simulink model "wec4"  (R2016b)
settings: Solver=ode4  StartTime=0  StopTime=1000  FixedStep=0.005  MaxStep=0.005  RelTol=1e-3  EnableMultiTasking=on
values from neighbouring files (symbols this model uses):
  arAdaptiveLawData = 1/2*zModelSimple.zModelPto.arFreq.*     zModelSimple.zModelPto.arMagnitude./     cos(zModelSimple.zModelPto.arPhase*pi/180+pi/2)    [IMPACT_Control.m]
  arAdaptiveLawDataX = 1/2*zModelSimpleX.zModelPto.arFreq.*         zModelSimpleX.zModelPto.arMagnitude./         cos(zModelSimpleX.zModelPto.arPhase*pi/180+pi/2)    [IMPACT_Control.m]
  arControllerRampGain = [0,0,1,1]    [IMPACT_Control.m]
  arControllerRampTime = [0 rStartRampTime rStartRampTime+rRampTimeLength 8000]    [IMPACT_Control.m]
  arEkfInitialisation = zeros(1,11)    [IMPACT_Control.m]
  arEkfInitialisationX = zeros(1,11)    [IMPACT_Control.m]
  arFrequency = zModelSimple.zModelPto.arFreq    [IMPACT_Control.m]
  arFrequencyRange = zModelSimple.zModelPto.arFreq    [IMPACT_Control.m]
  arFrequencyX = zModelSimpleX.zModelPto.arFreq    [IMPACT_Control.m]
  arImpedance = 1./zModelSimple.zModelPto.arMagnitude./zModelSimple.zModelPto.arFreq    [IMPACT_Control.m]
  arImpedanceX = 1./zModelSimpleX.zModelPto.arMagnitude./zModelSimpleX.zModelPto.arFreq    [IMPACT_Control.m]
  CentralPTOPreload = -1.6113e+07    (= -16113000)    [wecSimInputFile.m]
  F1 = [4.243 2.375 -12.243]    [wecSimInputFile.m]
  F2 = [4.243 -2.375 -12.243]    [wecSimInputFile.m]
  F3 = [-4.243 -2.375 -12.243]    [wecSimInputFile.m]
  F4 = [-4.243 2.375 -12.243]    [wecSimInputFile.m]
  FC = [0 0 -14]    [wecSimInputFile.m]
  iAdaptiveDamping = 0    [wec4IMPACT_Project.m]    (also in IMPACT_Control.m = handles.iAdaptiveDamping; wec1_IMPACT_Project.m; wec2_IMPACT_Project.m; wec3_IMPACT_Project.m)
  iControlType = 2    [wec4IMPACT_Project.m]    (also in IMPACT_Control.m = handles.iControlType; wec1_IMPACT_Project.m = 1; wec2_IMPACT_Project.m = 1; wec3_IMPACT_Project.m = 1)
  iPtoPositionConstraint = 1    [wec4IMPACT_Project.m]    (also in IMPACT_Control.m = handles.iPtoPositionConstraint; wec1_IMPACT_Project.m = 0; wec2_IMPACT_Project.m; wec3_IMPACT_Project.m)
  iSensorNoise = 0    [IMPACT_Control.m]
  m = m+1    (= 2)    [checkParamFile.m]
  PTOrotation = atan((T1(2)-F1(2))/(T1(1)-F1(1)))    [wecSimInputFile.m]
  rCogFloater = -8    [wec4_IMPACT_Model.m]    (also in paramInitial.m = get( handles.edit_rCogFloater, 'String' ); wec1_IMPACT_Model.m = -18; wec2_IMPACT_Model.m = -8.5; wec3_IMPACT_Model.m = -0.7)
  rCogSpar = -36.6    [wec4_IMPACT_Model.m]    (also in paramInitial.m = get( handles.edit_rCogSpar, 'String' ); wec3_IMPACT_Model.m = -21.3; wec3_IMPACT_Model2.m = -21.3)
  rDisplacementLimit = 10.000000    (= 10)    [wec4IMPACT_Project.m]    (also in IMPACT_Control.m = getValue(handles.edit_displacementLimit); wec1_IMPACT_Project.m; wec2_IMPACT_Project.m; wec3_IMPACT_Project.m = 3)
  rDisplacementLimitX = 10.000000    (= 10)    [wec4IMPACT_Project.m]    (also in IMPACT_Control.m = getValue(handles.edit_displacementLimitX); wec1_IMPACT_Project.m = 0; wec2_IMPACT_Project.m; wec3_IMPACT_Project.m = 0)
  rGainForAntiWIndUp = tfControllerDiscrete.rGain    [IMPACT_Control.m]
  rGainForAntiWIndUpX = tfControllerXDiscrete.rGain    [IMPACT_Control.m]
  rMaxForcePto = 300000000.000000    (= 300000000)    [wec4IMPACT_Project.m]    (also in IMPACT_Control.m = getValue(handles.edit_maxForcePto); wec1_IMPACT_Project.m = 1e+15; wec2_IMPACT_Project.m = 1e+15; wec3_IMPACT_Project.m = 1000000000)
  rMinForcePto = -300000000.000000    (= -300000000)    [wec4IMPACT_Project.m]    (also in IMPACT_Control.m = getValue(handles.edit_minForcePto); wec1_IMPACT_Project.m = -1e+15; wec2_IMPACT_Project.m = -1e+15; wec3_IMPACT_Project.m = -1000000000)
  rMooringX = 20000    [wec4_IMPACT_Model.m]    (also in paramInitial.m = get( handles.edit_rMooringX, 'String' ); wec3_IMPACT_Model.m = 10000; wec3_IMPACT_Model2.m = 10000)
  rMooringZ = 10000    [wec4_IMPACT_Model.m]    (also in paramInitial.m = get( handles.edit_rMooringZ, 'String' ); wec3_IMPACT_Model.m = 0; wec3_IMPACT_Model2.m = 0)
  rOutputSampleTime = 0.010000    (= 0.01)    [wec4IMPACT_Project.m]    (also in IMPACT_Control.m = getValue(handles.edit_outputSampleTime); wec1_IMPACT_Project.m; wec2_IMPACT_Project.m; wec3_IMPACT_Project.m)
  rPassiveDampingGain = -604830.000000    (= -604830)    [wec4IMPACT_Project.m]    (also in IMPACT_Control.m = getValue(handles.edit_gainPLD); wec1_IMPACT_Project.m = -214018.1537; wec2_IMPACT_Project.m = -1948070; wec3_IMPACT_Project.m = -519390)
  rPassiveDampingGainX = -278660.000000    (= -278660)    [wec4IMPACT_Project.m]    (also in IMPACT_Control.m = getValue(handles.edit_gainPLDX); wec1_IMPACT_Project.m = 0; wec2_IMPACT_Project.m = 0; wec3_IMPACT_Project.m = 0)
  rTetherPretension = 1.6113e+07    (= 16113000)    [wec4_IMPACT_Model.m]    (also in paramInitial.m = get( handles.edit_rTetherPretension, 'String' ); wec3_IMPACT_Model.m = 0; wec3_IMPACT_Model2.m = 0)
  rTetherSpring = 500000    [wec4_IMPACT_Model.m]    (also in paramInitial.m = get( handles.edit_rTetherSpring, 'String' ); wec3_IMPACT_Model.m = 0; wec3_IMPACT_Model2.m = 0)
  rUpperFrequencyLimit = EKFFloater.upperFreq    [IMPACT_Control.m]
  rXf = 4.243    [wec4AdditionalParams.m]
  rXs = 16.075    [wec4AdditionalParams.m]
  rYf = 2.375    [wec4AdditionalParams.m]
  rYs = 16.075    [wec4AdditionalParams.m]
  rZf = 4.243    [wec4AdditionalParams.m]
  rZs = 2.4350    (= 2.435)    [wec4AdditionalParams.m]
  rZTetherF = 6    [wec4AdditionalParams.m]
  rZTetherS = 2.4350    (= 2.435)    [wec4AdditionalParams.m]
  s = tf('s')    [wec4_IMPACT_Model.m]    (also in IMPACT_Control.m; wec1_IMPACT_Model.m; wec2_IMPACT_Model.m; wec3_IMPACT_Model.m)
  SidePTO1Preload = PreloadPTOCorner    (= 0)    [wecSimInputFile.m]
  SidePTO2Preload = PreloadPTOCorner    (= 0)    [wecSimInputFile.m]
  SidePTO3Preload = PreloadPTOCorner    (= 0)    [wecSimInputFile.m]
  SidePTO4Preload = PreloadPTOCorner    (= 0)    [wecSimInputFile.m]
  simu = simulationClass()    [wecSimInputFile.m]
  T1 = [16.075 16.075 -34.165]    [wecSimInputFile.m]
  T2 = [16.075 -16.075 -34.165]    [wecSimInputFile.m]
  T3 = [-16.075 -16.075 -34.165]    [wecSimInputFile.m]
  T4 = [-16.075 16.075 -34.165]    [wecSimInputFile.m]
  TC = [0 0 -34.165]    [wecSimInputFile.m]
  waves = waveClass('irregular')    [wecSimInputFile.m]
  Z = magPhaseToComplex(zModelTf)    [IMPACT_Control.m]
undefined symbols (not defined in the file or in its folder): arControllerDiscreteDen, arControllerDiscreteNum, arControllerDiscreteXDen, arControllerDiscreteXNum, arExcForceFloaterDen, arExcForceFloaterNum, arExcForceFloaterXDen, arExcForceFloaterXNum, arExcForceSparDen, arExcForceSparNum, arExcForceSparXDen, arExcForceSparXNum, arFexcFloaterDen, arFexcFloaterNum, arFexcFloaterXDen, arFexcFloaterXNum, arFexcSparDen, arFexcSparNum, arFexcSparXDen, arFexcSparXNum, Body, body, constraint, CTTime, deg, Elements, geometry, IRKB, kg, lenJ, mooring, N, pto, rAccelerationGainFloater, rAccelerationGainFloaterX, rAccelerationGainSpar, rAccelerationGainSparX, rad, rBuoyancyGainFloater, rBuoyancyGainFloaterX, rBuoyancyGainSpar, rBuoyancyGainSparX, rDampingGainFloater, rDampingGainFloaterX, rDampingGainSpar, rDampingGainSparX, Rigid, rMaxFocePto, wec4_float, wec4_reactor, WECSim_Lib, X, Y
libraries: nesl_utility x380, sm_lib x170, vrlib x91, simulink x12, WECSim_Lib x4
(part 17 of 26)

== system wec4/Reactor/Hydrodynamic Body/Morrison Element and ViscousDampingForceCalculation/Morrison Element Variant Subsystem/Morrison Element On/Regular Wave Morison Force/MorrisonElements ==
  r : Inport  Partition=on  PartitionDimension=1  PartitionWidth=1
  Vel : Inport  Port=2
  Accel : Inport  Port=3
  Disp : Inport  Port=4
  Area : Inport  Port=5  Partition=on  PartitionDimension=1  PartitionWidth=1
  Cd : Inport  Port=6  Partition=on  PartitionDimension=1  PartitionWidth=1
  Vol : Inport  Port=7  Partition=on  PartitionDimension=1  PartitionWidth=1
  Ca : Inport  Port=8  Partition=on  PartitionDimension=1  PartitionWidth=1
  Time : Inport  Port=9
  3x3 : Concatenate  NumInputs=3  Mode=Multidimensional array
  A x 3x3 : Product  Multiplication=Matrix(*)
  Accel-sl : Selector  InputPortWidth=6  IndexOptions=Index vector (dialog)  Indices=[1 2 3]  OutputSizes=1
  Accel-sr : Selector  InputPortWidth=6  IndexOptions=Index vector (dialog)  Indices=[4 5 6]  OutputSizes=1
  AccelDiff-u : Sum  Inputs=+-
  AccelDiff-v : Sum  Inputs=+-
  AccelDiff-w : Sum  Inputs=+-
  Add Accel : Sum  Inputs=+++
  Add Vel : Sum
  Ax : Selector  InputPortWidth=3  IndexOptions=Index vector (dialog)  Indices=[1]  OutputSizes=1
  Ay : Selector  InputPortWidth=3  IndexOptions=Index vector (dialog)  Indices=[2]  OutputSizes=1
  Az : Selector  InputPortWidth=3  IndexOptions=Index vector (dialog)  Indices=[3]  OutputSizes=1
  Cax : Selector  InputPortWidth=3  IndexOptions=Index vector (dialog)  Indices=[1]  OutputSizes=1
  Cay : Selector  InputPortWidth=3  IndexOptions=Index vector (dialog)  Indices=[2]  OutputSizes=1
  Caz : Selector  InputPortWidth=3  IndexOptions=Index vector (dialog)  Indices=[3]  OutputSizes=1
  Cdx : Selector  InputPortWidth=3  IndexOptions=Index vector (dialog)  Indices=[1]  OutputSizes=1
  Cdy : Selector  InputPortWidth=3  IndexOptions=Index vector (dialog)  Indices=[2]  OutputSizes=1
  Cdz : Selector  InputPortWidth=3  IndexOptions=Index vector (dialog)  Indices=[3]  OutputSizes=1
  Constant : Constant  Value=0
  Density : Constant  Value=simu.rho
  Disp-sl : Selector  InputPortWidth=6  IndexOptions=Index vector (dialog)  Indices=[1 2 3]  OutputSizes=1
  Disp-sr : Selector  InputPortWidth=6  IndexOptions=Index vector (dialog)  Indices=[4 5 6]  OutputSizes=1
  For Each : ForEach  DisableCoverage=on  IndexMode=One-based
  ForceCom : Concatenate  NumInputs=3  ConcatenateDimension=2
  Fout : Concatenate  NumInputs=6  Mode=Multidimensional array  ConcatenateDimension=2
  Fx-A : Product  Inputs=4
  Fx-AFK : Product  Inputs=3
  Fx-Sum : Sum  Inputs=+++
  Fx-V : Product  Inputs=5
  Fx-V1 : Product  Inputs=5
  Fy-A : Product  Inputs=4
  Fy-AFK : Product  Inputs=3
  Fy-Sum : Sum  Inputs=+++
  Fz-A : Product  Inputs=4
  Fz-AFK : Product  Inputs=3
  Fz-Sum : Sum  Inputs=+++
  Fz-w : Product  Inputs=5
  Mx : Selector  InputPortWidth=3  IndexOptions=Index vector (dialog)  Indices=[1]  OutputSizes=1
  My : Selector  InputPortWidth=3  IndexOptions=Index vector (dialog)  Indices=[2]  OutputSizes=1
  Mz : Selector  InputPortWidth=3  IndexOptions=Index vector (dialog)  Indices=[3]  OutputSizes=1
  OrbitalVelocity : Subsystem
  Rotation1 : Subsystem
  Rotation2 : Subsystem
  Rotation3 : Subsystem
  ShiftCg : Sum
  SwitchFx : Switch  Criteria=u2 > Threshold
  SwitchFy : Switch  Criteria=u2 > Threshold
  SwitchFz : Switch  Criteria=u2 > Threshold
  Ux : Selector  InputPortWidth=3  IndexOptions=Index vector (dialog)  Indices=[1]  OutputSizes=1
  Uy : Selector  InputPortWidth=3  IndexOptions=Index vector (dialog)  Indices=[2]  OutputSizes=1
  Uz : Selector  InputPortWidth=3  IndexOptions=Index vector (dialog)  Indices=[3]  OutputSizes=1
  V-u : Abs
  V-v : Abs
  V-w : Abs
  V^2-u : Product
  V^2-v : Product
  V^2-w : Product
  Vel-sl : Selector  InputPortWidth=6  IndexOptions=Index vector (dialog)  Indices=[1 2 3]  OutputSizes=1
  "Vel-sr " : Selector  InputPortWidth=6  IndexOptions=Index vector (dialog)  Indices=[4 5 6]  OutputSizes=1
  VelDiff-u : Sum  Inputs=+-
  VelDiff-v : Sum  Inputs=+-
  VelDiff-w : Sum  Inputs=+-
  Zshift : Selector  InputPortWidth=3  IndexOptions=Index vector (dialog)  Indices=[3]  OutputSizes=1
  abs-Area : Abs
  abs-Ca : Abs
  abs-Cd : Abs
  "dot{U}x" : Selector  InputPortWidth=3  IndexOptions=Index vector (dialog)  Indices=[1]  OutputSizes=1
  "dot{U}y" : Selector  InputPortWidth=3  IndexOptions=Index vector (dialog)  Indices=[2]  OutputSizes=1
  "dot{U}z" : Selector  InputPortWidth=3  IndexOptions=Index vector (dialog)  Indices=[3]  OutputSizes=1
  "dot{w} x r2" : vrlib/Utilities/Cross Product
  half : Constant  Value=1/2
  r x 3x1 : Product  Multiplication=Matrix(*)
  r x 3x2 : Product  Multiplication=Matrix(*)
  r x 3x3 : Product  Multiplication=Matrix(*)
  "r_{cg} x F" : vrlib/Utilities/Cross Product
  rot1 : Selector  InputPortWidth=3  IndexOptions=Index vector (dialog)  Indices=[1]  OutputSizes=1
  rot2 : Selector  InputPortWidth=3  IndexOptions=Index vector (dialog)  Indices=[2]  OutputSizes=1
  rot3 : Selector  InputPortWidth=3  IndexOptions=Index vector (dialog)  Indices=[3]  OutputSizes=1
  w x r : vrlib/Utilities/Cross Product
  w x w x r : vrlib/Utilities/Cross Product
  Force : Outport  PortDimensions=[1 6]  ConcatenationDimension=1
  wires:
  Time/1 -> OrbitalVelocity/2(Time)
  abs-Cd/1 -> r x 3x1/1
  abs-Ca/1 -> Caz/1, Cay/1, Cax/1
  V-w/1 -> V^2-w/1
  Constant/1 -> SwitchFx/1, SwitchFz/1, SwitchFy/1
  Fx-V1/1 -> Fy-Sum/1
  Fy-A/1 -> Fy-Sum/2
  Cay/1 -> Fy-A/4
  AccelDiff-v/1 -> Fy-A/1
  Fy-AFK/1 -> Fy-Sum/3
  Fy-Sum/1 -> SwitchFy/3
  SwitchFy/1 -> ForceCom/2, Fout/2
  Cdy/1 -> Fx-V1/4
  Ay/1 -> Fx-V1/5
  OrbitalVelocity/5(v-V) -> VelDiff-v/1
  VelDiff-v/1 -> V^2-v/2, V-v/1
  V-v/1 -> V^2-v/1
  V^2-v/1 -> Fx-V1/1
  OrbitalVelocity/6(v-A) -> Fy-AFK/1, AccelDiff-v/1
  r x 3x2/1 -> abs-Ca/1
  Ca/1 -> r x 3x2/1
  r x 3x1/1 -> Cdx/1, Cdz/1, Cdy/1
  Cd/1 -> abs-Cd/1
  Cax/1 -> Fx-A/4
  Caz/1 -> Fz-A/4
  Fout/1 -> Force/1
  ForceCom/1 -> "r_{cg} x F"/2
  abs-Area/1 -> Ax/1, Az/1, Ay/1
  A x 3x3/1 -> abs-Area/1
  Cdz/1 -> Fz-w/4
  Cdx/1 -> Fx-V/4
  Ax/1 -> Fx-V/5
  Area/1 -> A x 3x3/1
  Az/1 -> Fz-w/5
  Fz-Sum/1 -> SwitchFz/3
  Fx-Sum/1 -> SwitchFx/3
  SwitchFx/1 -> ForceCom/1, Fout/1
  SwitchFz/1 -> Fout/3, ForceCom/3
  Zshift/1 -> SwitchFz/2, SwitchFx/2, SwitchFy/2
  VelDiff-u/1 -> V^2-u/2, V-u/1
  V-u/1 -> V^2-u/1
  3x3/1 -> r x 3x1/2, r x 3x2/2, r x 3x3/2, A x 3x3/2
  Mz/1 -> Fout/6
  My/1 -> Fout/5
  Mx/1 -> Fout/4
  "r_{cg} x F"/1 -> Mx/1, My/1, Mz/1
  Fz-AFK/1 -> Fz-Sum/3
  Fz-A/1 -> Fz-Sum/2
  Fz-w/1 -> Fz-Sum/1
  Fx-AFK/1 -> Fx-Sum/3
  Fx-A/1 -> Fx-Sum/2
  Fx-V/1 -> Fx-Sum/1
  OrbitalVelocity/4(w-A) -> AccelDiff-w/1, Fz-AFK/1
  AccelDiff-w/1 -> Fz-A/1
  Vol/1 -> Fx-A/3, Fz-A/2, Fx-AFK/2, Fz-AFK/2, Fy-AFK/2, Fy-A/2
  AccelDiff-u/1 -> Fx-A/1
  V^2-w/1 -> Fz-w/1
  Density/1 -> Fx-V/3, Fx-V1/3, Fz-w/3, Fx-A/2, Fz-A/3, Fx-AFK/3, Fz-AFK/3, Fy-AFK/3, Fy-A/3
  half/1 -> Fx-V/2, Fx-V1/2, Fz-w/2
  V^2-u/1 -> Fx-V/1
  VelDiff-w/1 -> V^2-w/2, V-w/1
  OrbitalVelocity/2(w-V) -> VelDiff-w/1
  OrbitalVelocity/1(u-V) -> VelDiff-u/1
  Uz/1 -> VelDiff-w/2
  Ux/1 -> VelDiff-u/2
  Uy/1 -> VelDiff-v/2
  Add Vel/1 -> Ux/1, Uz/1, Uy/1
  "dot{U}z"/1 -> AccelDiff-w/2
  OrbitalVelocity/3(u-A) -> Fx-AFK/1, AccelDiff-u/1
  "dot{U}x"/1 -> AccelDiff-u/2
  "dot{U}y"/1 -> AccelDiff-v/2
  ShiftCg/1 -> OrbitalVelocity/1(Disp), Zshift/1
  Disp-sl/1 -> ShiftCg/2
  r x 3x3/1 -> ShiftCg/1, "r_{cg} x F"/1
  Rotation3/1(rot[3,1-3]) -> 3x3/3
  Rotation1/1(rot[1,1-3]) -> 3x3/1
  Rotation2/1(rot[2,1-3]) -> 3x3/2
  rot2/1 -> Rotation1/2(rot2), Rotation2/2(rot2), Rotation3/2(rot2)
  rot1/1 -> Rotation1/1(rot1), Rotation2/1(rot1), Rotation3/1(rot1)
  rot3/1 -> Rotation1/3(rot3), Rotation2/3(rot3)
  Disp-sr/1 -> rot1/1, rot2/1, rot3/1
  Disp/1 -> Disp-sr/1, Disp-sl/1
  Vel-sl/1 -> Add Vel/1
  Add Accel/1 -> "dot{U}x"/1, "dot{U}y"/1, "dot{U}z"/1
  Accel-sl/1 -> Add Accel/3
  "dot{w} x r2"/1 -> Add Accel/2
  Accel-sr/1 -> "dot{w} x r2"/1
  Accel/1 -> Accel-sr/1, Accel-sl/1
  r/1 -> w x r/2, "dot{w} x r2"/2, r x 3x3/1
  "Vel-sr "/1 -> w x r/1, w x w x r/1
  w x w x r/1 -> Add Accel/1
  w x r/1 -> w x w x r/2, Add Vel/2
  Vel/1 -> "Vel-sr "/1, Vel-sl/1

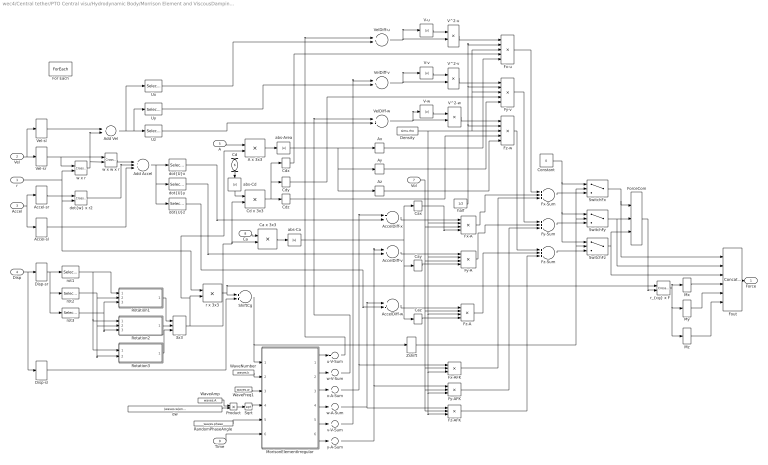
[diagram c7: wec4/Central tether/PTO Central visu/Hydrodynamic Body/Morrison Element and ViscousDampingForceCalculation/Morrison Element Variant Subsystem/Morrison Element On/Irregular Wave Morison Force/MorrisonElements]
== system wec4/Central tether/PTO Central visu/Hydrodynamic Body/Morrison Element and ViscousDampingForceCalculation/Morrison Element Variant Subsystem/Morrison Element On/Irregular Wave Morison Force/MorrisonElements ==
  r : Inport  Partition=on  PartitionDimension=1  PartitionWidth=1
  Vel : Inport  Port=2
  Accel : Inport  Port=3
  Disp : Inport  Port=4
  A : Inport  Port=5  Partition=on  PartitionDimension=1  PartitionWidth=1
  Cd : Inport  Port=6  Partition=on  PartitionDimension=1  PartitionWidth=1
  Vol : Inport  Port=7  Partition=on  PartitionDimension=1  PartitionWidth=1
  Ca : Inport  Port=8  Partition=on  PartitionDimension=1  PartitionWidth=1
  Time : Inport  Port=9
  3x3 : Concatenate  NumInputs=3  Mode=Multidimensional array
  A x 3x3 : Product  Multiplication=Matrix(*)
  Accel-sl : Selector  InputPortWidth=6  IndexOptions=Index vector (dialog)  Indices=[1 2 3]  OutputSizes=1
  Accel-sr : Selector  InputPortWidth=6  IndexOptions=Index vector (dialog)  Indices=[4 5 6]  OutputSizes=1
  AccelDiff-v : Sum  Inputs=+-
  AccelDiff-w : Sum  Inputs=+-
  AccelDiff-x : Sum  Inputs=+-
  Add Accel : Sum  Inputs=+++
  Add Vel : Sum
  Ax : Selector  InputPortWidth=3  IndexOptions=Index vector (dialog)  Indices=[1]  OutputSizes=1
  Ay : Selector  InputPortWidth=3  IndexOptions=Index vector (dialog)  Indices=[2]  OutputSizes=1
  Az : Selector  InputPortWidth=3  IndexOptions=Index vector (dialog)  Indices=[3]  OutputSizes=1
  Ca x 3x3 : Product  Multiplication=Matrix(*)
  Cax : Selector  InputPortWidth=3  IndexOptions=Index vector (dialog)  Indices=[1]  OutputSizes=1
  Cay : Selector  InputPortWidth=3  IndexOptions=Index vector (dialog)  Indices=[2]  OutputSizes=1
  Caz : Selector  InputPortWidth=3  IndexOptions=Index vector (dialog)  Indices=[3]  OutputSizes=1
  Cd x 3x3 : Product  Multiplication=Matrix(*)
  Cdx : Selector  InputPortWidth=3  IndexOptions=Index vector (dialog)  Indices=[1]  OutputSizes=1
  Cdy : Selector  InputPortWidth=3  IndexOptions=Index vector (dialog)  Indices=[2]  OutputSizes=1
  Cdz : Selector  InputPortWidth=3  IndexOptions=Index vector (dialog)  Indices=[3]  OutputSizes=1
  Constant : Constant  Value=0
  Density : Constant  Value=simu.rho
  Disp-sl : Selector  InputPortWidth=6  IndexOptions=Index vector (dialog)  Indices=[1 2 3]  OutputSizes=1
  Disp-sr : Selector  InputPortWidth=6  IndexOptions=Index vector (dialog)  Indices=[4 5 6]  OutputSizes=1
  For Each : ForEach  DisableCoverage=on  IndexMode=One-based
  ForceCom : Concatenate  NumInputs=3  ConcatenateDimension=2
  Fout : Concatenate  NumInputs=6  Mode=Multidimensional array  ConcatenateDimension=2
  Fx-A : Product  Inputs=4
  Fx-AFK : Product  Inputs=3
  Fx-Sum : Sum  Inputs=+++
  Fx-u : Product  Inputs=5
  Fy-A : Product  Inputs=4
  Fy-AFK : Product  Inputs=3
  Fy-Sum : Sum  Inputs=+++
  Fy-v : Product  Inputs=5
  Fz-A : Product  Inputs=4
  Fz-AFK : Product  Inputs=3
  Fz-Sum : Sum  Inputs=+++
  Fz-w : Product  Inputs=5
  MorisonElementIrregular : Subsystem  TreatAsAtomicUnit=on
  Mx : Selector  InputPortWidth=3  IndexOptions=Index vector (dialog)  Indices=[1]  OutputSizes=1
  My : Selector  InputPortWidth=3  IndexOptions=Index vector (dialog)  Indices=[2]  OutputSizes=1
  Mz : Selector  InputPortWidth=3  IndexOptions=Index vector (dialog)  Indices=[3]  OutputSizes=1
  Product : Product
  RandomPhaseAngle : Constant  Value=waves.phase  VectorParams1D=off
  Rotation1 : Subsystem
  Rotation2 : Subsystem
  Rotation3 : Subsystem
  ShiftCg : Sum
  Sqrt : Sqrt
  SwitchFx : Switch  Criteria=u2 > Threshold
  SwitchFy : Switch  Criteria=u2 > Threshold
  SwitchFz : Switch  Criteria=u2 > Threshold
  Ux : Selector  InputPortWidth=3  IndexOptions=Index vector (dialog)  Indices=[1]  OutputSizes=1
  Uy : Selector  InputPortWidth=3  IndexOptions=Index vector (dialog)  Indices=[2]  OutputSizes=1
  Uz : Selector  InputPortWidth=3  IndexOptions=Index vector (dialog)  Indices=[3]  OutputSizes=1
  V-u : Abs
  V-v : Abs
  V-w : Abs
  V^2-u : Product
  V^2-v : Product
  V^2-w : Product
  Vel-sl : Selector  InputPortWidth=6  IndexOptions=Index vector (dialog)  Indices=[1 2 3]  OutputSizes=1
  "Vel-sr " : Selector  InputPortWidth=6  IndexOptions=Index vector (dialog)  Indices=[4 5 6]  OutputSizes=1
  VelDiff-u : Sum  Inputs=+-
  VelDiff-v : Sum  Inputs=+-
  VelDiff-w : Sum  Inputs=+-
  WaveAmp : Constant  Value=waves.A  VectorParams1D=off
  WaveFreq1 : Constant  Value=waves.w  VectorParams1D=off
  WaveNumber : Constant  Value=waves.k  VectorParams1D=off
  Zshift : Selector  InputPortWidth=3  IndexOptions=Index vector (dialog)  Indices=[3]  OutputSizes=1
  abs-Area : Abs
  abs-Ca : Abs
  abs-Cd : Abs
  "dot{U}x" : Selector  InputPortWidth=3  IndexOptions=Index vector (dialog)  Indices=[1]  OutputSizes=1
  "dot{U}y" : Selector  InputPortWidth=3  IndexOptions=Index vector (dialog)  Indices=[2]  OutputSizes=1
  "dot{U}z" : Selector  InputPortWidth=3  IndexOptions=Index vector (dialog)  Indices=[3]  OutputSizes=1
  "dot{w} x r2" : vrlib/Utilities/Cross Product
  dw : Constant  Value=(waves.w(end)-waves.w(1))/(waves.numFreq-1)  VectorParams1D=off
  half : Constant  Value=1/2
  r x 3x3 : Product  Multiplication=Matrix(*)
  "r_{cg} x F" : vrlib/Utilities/Cross Product
  rot1 : Selector  InputPortWidth=3  IndexOptions=Index vector (dialog)  Indices=[1]  OutputSizes=1
  rot2 : Selector  InputPortWidth=3  IndexOptions=Index vector (dialog)  Indices=[2]  OutputSizes=1
  rot3 : Selector  InputPortWidth=3  IndexOptions=Index vector (dialog)  Indices=[3]  OutputSizes=1
  u-V-Sum : Sum  Inputs=+  CollapseMode=Specified dimension
  v-V-Sum : Sum  Inputs=+  CollapseMode=Specified dimension
  w x r : vrlib/Utilities/Cross Product
  w x w x r : vrlib/Utilities/Cross Product
  w-A-Sum : Sum  Inputs=+  CollapseMode=Specified dimension
  w-V-Sum : Sum  Inputs=+  CollapseMode=Specified dimension
  x-A-Sum : Sum  Inputs=+  CollapseMode=Specified dimension
  y-A-Sum : Sum  Inputs=+  CollapseMode=Specified dimension
  Force : Outport  PortDimensions=[1 6]  ConcatenationDimension=1
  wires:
  Time/1 -> MorisonElementIrregular/6(Time)
  abs-Cd/1 -> Cd x 3x3/1
  abs-Ca/1 -> Cay/1, Caz/1, Cax/1
  Fy-AFK/1 -> Fy-Sum/3
  Fy-A/1 -> Fy-Sum/2
  AccelDiff-v/1 -> Fy-A/1
  Cay/1 -> Fy-A/4
  y-A-Sum/1 -> AccelDiff-v/1, Fy-AFK/1
  Fy-v/1 -> Fy-Sum/1
  Fy-Sum/1 -> SwitchFy/3
  SwitchFy/1 -> ForceCom/2, Fout/2
  Cdy/1 -> Fy-v/4
  Ay/1 -> Fy-v/5
  V^2-v/1 -> Fy-v/1
  v-V-Sum/1 -> VelDiff-v/1
  V-v/1 -> V^2-v/1
  VelDiff-v/1 -> V^2-v/2, V-v/1
  V-w/1 -> V^2-w/1
  MorisonElementIrregular/6(y-A) -> y-A-Sum/1
  MorisonElementIrregular/5(v-V) -> v-V-Sum/1
  V-u/1 -> V^2-u/1
  MorisonElementIrregular/4(w-A) -> w-A-Sum/1
  MorisonElementIrregular/3(x-A) -> x-A-Sum/1
  MorisonElementIrregular/2(w-V) -> w-V-Sum/1
  Sqrt/1 -> MorisonElementIrregular/4(waves.A)
  Product/1 -> Sqrt/1
  dw/1 -> Product/2
  WaveAmp/1 -> Product/1
  MorisonElementIrregular/1(u-V) -> u-V-Sum/1
  RandomPhaseAngle/1 -> MorisonElementIrregular/5(waves.Phase)
  WaveFreq1/1 -> MorisonElementIrregular/3(waves.w)
  WaveNumber/1 -> MorisonElementIrregular/2(waves.kirr)
  Ca x 3x3/1 -> abs-Ca/1
  Ca/1 -> Ca x 3x3/1
  Cd x 3x3/1 -> Cdx/1, Cdy/1, Cdz/1
  Cd/1 -> abs-Cd/1
  Cax/1 -> Fx-A/4
  Caz/1 -> Fz-A/4
  Fout/1 -> Force/1
  ForceCom/1 -> "r_{cg} x F"/2
  abs-Area/1 -> Ax/1, Az/1, Ay/1
  A x 3x3/1 -> abs-Area/1
  Cdz/1 -> Fz-w/4
  Cdx/1 -> Fx-u/4
  Ax/1 -> Fx-u/5
  A/1 -> A x 3x3/1
  Az/1 -> Fz-w/5
  Fz-Sum/1 -> SwitchFz/3
  Fx-Sum/1 -> SwitchFx/3
  SwitchFx/1 -> ForceCom/1, Fout/1
  SwitchFz/1 -> Fout/3, ForceCom/3
  Zshift/1 -> SwitchFz/2, SwitchFx/2, SwitchFy/2
  VelDiff-u/1 -> V^2-u/2, V-u/1
  3x3/1 -> Cd x 3x3/2, Ca x 3x3/2, r x 3x3/2, A x 3x3/2
  Mz/1 -> Fout/6
  My/1 -> Fout/5
  Mx/1 -> Fout/4
  "r_{cg} x F"/1 -> Mx/1, My/1, Mz/1
  Constant/1 -> SwitchFx/1, SwitchFz/1, SwitchFy/1
  Fz-AFK/1 -> Fz-Sum/3
  Fz-A/1 -> Fz-Sum/2
  Fz-w/1 -> Fz-Sum/1
  Fx-AFK/1 -> Fx-Sum/3
  Fx-A/1 -> Fx-Sum/2
  Fx-u/1 -> Fx-Sum/1
  w-A-Sum/1 -> Fz-AFK/1, AccelDiff-w/1
  AccelDiff-w/1 -> Fz-A/1
  Vol/1 -> Fx-A/3, Fz-A/2, Fx-AFK/2, Fz-AFK/2, Fy-AFK/2, Fy-A/3
  AccelDiff-x/1 -> Fx-A/1
  V^2-w/1 -> Fz-w/1
  Density/1 -> Fz-w/3, Fx-u/3, Fy-v/3, Fx-A/2, Fz-A/3, Fx-AFK/3, Fz-AFK/3, Fy-AFK/3, Fy-A/2
  half/1 -> Fx-u/2, Fy-v/2, Fz-w/2
  V^2-u/1 -> Fx-u/1
  VelDiff-w/1 -> V-w/1, V^2-w/2
  w-V-Sum/1 -> VelDiff-w/1
  u-V-Sum/1 -> VelDiff-u/1
  Uz/1 -> VelDiff-w/2
  Ux/1 -> VelDiff-u/2
  Uy/1 -> VelDiff-v/2
  Add Vel/1 -> Uz/1, Uy/1, Ux/1
  "dot{U}z"/1 -> AccelDiff-w/2
  x-A-Sum/1 -> AccelDiff-x/1, Fx-AFK/1
  "dot{U}x"/1 -> AccelDiff-x/2
  "dot{U}y"/1 -> AccelDiff-v/2
  ShiftCg/1 -> Zshift/1, MorisonElementIrregular/1(Disp)
  Disp-sl/1 -> ShiftCg/2
  r x 3x3/1 -> ShiftCg/1, "r_{cg} x F"/1
  Rotation3/1(rot[3,1-3]) -> 3x3/3
  Rotation1/1(rot[1,1-3]) -> 3x3/1
  Rotation2/1(rot[2,1-3]) -> 3x3/2
  rot2/1 -> Rotation1/2(rot2), Rotation2/2(rot2), Rotation3/2(rot2)
  rot1/1 -> Rotation1/1(rot1), Rotation2/1(rot1), Rotation3/1(rot1)
  rot3/1 -> Rotation1/3(rot3), Rotation2/3(rot3)
  Disp-sr/1 -> rot1/1, rot2/1, rot3/1
  Disp/1 -> Disp-sr/1, Disp-sl/1
  Vel-sl/1 -> Add Vel/1
  Add Accel/1 -> "dot{U}x"/1, "dot{U}y"/1, "dot{U}z"/1
  Accel-sl/1 -> Add Accel/3
  "dot{w} x r2"/1 -> Add Accel/2
  Accel-sr/1 -> "dot{w} x r2"/1
  Accel/1 -> Accel-sr/1, Accel-sl/1
  r/1 -> w x r/2, "dot{w} x r2"/2, r x 3x3/1
  "Vel-sr "/1 -> w x r/1, w x w x r/1
  w x w x r/1 -> Add Accel/1
  w x r/1 -> w x w x r/2, Add Vel/2
  Vel/1 -> "Vel-sr "/1, Vel-sl/1

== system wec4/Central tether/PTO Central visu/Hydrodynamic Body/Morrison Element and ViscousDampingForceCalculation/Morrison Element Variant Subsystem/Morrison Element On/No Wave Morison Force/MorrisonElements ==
  r : Inport  Partition=on  PartitionDimension=1  PartitionWidth=1
  Vel : Inport  Port=2
  Accel : Inport  Port=3
  Disp : Inport  Port=4
  Area : Inport  Port=5  Partition=on  PartitionDimension=1  PartitionWidth=1
  Cd : Inport  Port=6  Partition=on  PartitionDimension=1  PartitionWidth=1
  Vol : Inport  Port=7  Partition=on  PartitionDimension=1  PartitionWidth=1
  Ca : Inport  Port=8  Partition=on  PartitionDimension=1  PartitionWidth=1
  Time : Inport  Port=9
  3x3 : Concatenate  NumInputs=3  Mode=Multidimensional array
  A x 3x3 : Product  Multiplication=Matrix(*)
  Accel-sl : Selector  InputPortWidth=6  IndexOptions=Index vector (dialog)  Indices=[1 2 3]  OutputSizes=1
  Accel-sr : Selector  InputPortWidth=6  IndexOptions=Index vector (dialog)  Indices=[4 5 6]  OutputSizes=1
  AccelDiff-u : Sum  Inputs=+-
  AccelDiff-v : Sum  Inputs=+-
  AccelDiff-w : Sum  Inputs=+-
  Add Accel : Sum  Inputs=+++
  Add Vel : Sum
  Ax : Selector  InputPortWidth=3  IndexOptions=Index vector (dialog)  Indices=[1]  OutputSizes=1
  Ay : Selector  InputPortWidth=3  IndexOptions=Index vector (dialog)  Indices=[2]  OutputSizes=1
  Az : Selector  InputPortWidth=3  IndexOptions=Index vector (dialog)  Indices=[3]  OutputSizes=1
  Cax : Selector  InputPortWidth=3  IndexOptions=Index vector (dialog)  Indices=[1]  OutputSizes=1
  Cay : Selector  InputPortWidth=3  IndexOptions=Index vector (dialog)  Indices=[2]  OutputSizes=1
  Caz : Selector  InputPortWidth=3  IndexOptions=Index vector (dialog)  Indices=[3]  OutputSizes=1
  Cdx : Selector  InputPortWidth=3  IndexOptions=Index vector (dialog)  Indices=[1]  OutputSizes=1
  Cdy : Selector  InputPortWidth=3  IndexOptions=Index vector (dialog)  Indices=[2]  OutputSizes=1
  Cdz : Selector  InputPortWidth=3  IndexOptions=Index vector (dialog)  Indices=[3]  OutputSizes=1
  Constant : Constant  Value=0
  Density : Constant  Value=simu.rho
  Disp-sl : Selector  InputPortWidth=6  IndexOptions=Index vector (dialog)  Indices=[1 2 3]  OutputSizes=1
  Disp-sr : Selector  InputPortWidth=6  IndexOptions=Index vector (dialog)  Indices=[4 5 6]  OutputSizes=1
  For Each : ForEach  DisableCoverage=on  IndexMode=One-based
  ForceCom : Concatenate  NumInputs=3  ConcatenateDimension=2
  Fout : Concatenate  NumInputs=6  Mode=Multidimensional array  ConcatenateDimension=2
  Fx-A : Product  Inputs=4
  Fx-AFK : Product  Inputs=3
  Fx-Sum : Sum  Inputs=+++
  Fx-V : Product  Inputs=5
  Fx-V1 : Product  Inputs=5
  Fy-A : Product  Inputs=4
  Fy-AFK : Product  Inputs=3
  Fy-Sum : Sum  Inputs=+++
  Fz-A : Product  Inputs=4
  Fz-AFK : Product  Inputs=3
  Fz-Sum : Sum  Inputs=+++
  Fz-w : Product  Inputs=5
  Mx : Selector  InputPortWidth=3  IndexOptions=Index vector (dialog)  Indices=[1]  OutputSizes=1
  My : Selector  InputPortWidth=3  IndexOptions=Index vector (dialog)  Indices=[2]  OutputSizes=1
  Mz : Selector  InputPortWidth=3  IndexOptions=Index vector (dialog)  Indices=[3]  OutputSizes=1
  OrbitalVelocity : Subsystem
  Rotation1 : Subsystem
  Rotation2 : Subsystem
  Rotation3 : Subsystem
  ShiftCg : Sum
  SwitchFx : Switch  Criteria=u2 > Threshold
  SwitchFy : Switch  Criteria=u2 > Threshold
  SwitchFz : Switch  Criteria=u2 > Threshold
  Ux : Selector  InputPortWidth=3  IndexOptions=Index vector (dialog)  Indices=[1]  OutputSizes=1
  Uy : Selector  InputPortWidth=3  IndexOptions=Index vector (dialog)  Indices=[2]  OutputSizes=1
  Uz : Selector  InputPortWidth=3  IndexOptions=Index vector (dialog)  Indices=[3]  OutputSizes=1
  V-u : Abs
  V-v : Abs
  V-w : Abs
  V^2-u : Product
  V^2-v : Product
  V^2-w : Product
  Vel-sl : Selector  InputPortWidth=6  IndexOptions=Index vector (dialog)  Indices=[1 2 3]  OutputSizes=1
  "Vel-sr " : Selector  InputPortWidth=6  IndexOptions=Index vector (dialog)  Indices=[4 5 6]  OutputSizes=1
  VelDiff-u : Sum  Inputs=+-
  VelDiff-v : Sum  Inputs=+-
  VelDiff-w : Sum  Inputs=+-
  Zshift : Selector  InputPortWidth=3  IndexOptions=Index vector (dialog)  Indices=[3]  OutputSizes=1
  abs-Area : Abs
  abs-Ca : Abs
  abs-Cd : Abs
  "dot{U}x" : Selector  InputPortWidth=3  IndexOptions=Index vector (dialog)  Indices=[1]  OutputSizes=1
  "dot{U}y" : Selector  InputPortWidth=3  IndexOptions=Index vector (dialog)  Indices=[2]  OutputSizes=1
  "dot{U}z" : Selector  InputPortWidth=3  IndexOptions=Index vector (dialog)  Indices=[3]  OutputSizes=1
  "dot{w} x r2" : vrlib/Utilities/Cross Product
  half : Constant  Value=1/2
  r x 3x1 : Product  Multiplication=Matrix(*)
  r x 3x2 : Product  Multiplication=Matrix(*)
  r x 3x3 : Product  Multiplication=Matrix(*)
  "r_{cg} x F" : vrlib/Utilities/Cross Product
  rot1 : Selector  InputPortWidth=3  IndexOptions=Index vector (dialog)  Indices=[1]  OutputSizes=1
  rot2 : Selector  InputPortWidth=3  IndexOptions=Index vector (dialog)  Indices=[2]  OutputSizes=1
  rot3 : Selector  InputPortWidth=3  IndexOptions=Index vector (dialog)  Indices=[3]  OutputSizes=1
  w x r : vrlib/Utilities/Cross Product
  w x w x r : vrlib/Utilities/Cross Product
  Force : Outport  PortDimensions=[1 6]  ConcatenationDimension=1
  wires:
  Time/1 -> OrbitalVelocity/2(Time)
  abs-Cd/1 -> r x 3x1/1
  abs-Ca/1 -> Caz/1, Cay/1, Cax/1
  V-w/1 -> V^2-w/1
  Constant/1 -> SwitchFx/1, SwitchFz/1, SwitchFy/1
  Fx-V1/1 -> Fy-Sum/1
  Fy-A/1 -> Fy-Sum/2
  Cay/1 -> Fy-A/4
  AccelDiff-v/1 -> Fy-A/1
  Fy-AFK/1 -> Fy-Sum/3
  Fy-Sum/1 -> SwitchFy/3
  SwitchFy/1 -> ForceCom/2, Fout/2
  Cdy/1 -> Fx-V1/4
  Ay/1 -> Fx-V1/5
  OrbitalVelocity/5(v-V) -> VelDiff-v/1
  VelDiff-v/1 -> V^2-v/2, V-v/1
  V-v/1 -> V^2-v/1
  V^2-v/1 -> Fx-V1/1
  OrbitalVelocity/6(v-A) -> Fy-AFK/1, AccelDiff-v/1
  r x 3x2/1 -> abs-Ca/1
  Ca/1 -> r x 3x2/1
  r x 3x1/1 -> Cdx/1, Cdz/1, Cdy/1
  Cd/1 -> abs-Cd/1
  Cax/1 -> Fx-A/4
  Caz/1 -> Fz-A/4
  Fout/1 -> Force/1
  ForceCom/1 -> "r_{cg} x F"/2
  abs-Area/1 -> Ax/1, Az/1, Ay/1
  A x 3x3/1 -> abs-Area/1
  Cdz/1 -> Fz-w/4
  Cdx/1 -> Fx-V/4
  Ax/1 -> Fx-V/5
  Area/1 -> A x 3x3/1
  Az/1 -> Fz-w/5
  Fz-Sum/1 -> SwitchFz/3
  Fx-Sum/1 -> SwitchFx/3
  SwitchFx/1 -> ForceCom/1, Fout/1
  SwitchFz/1 -> Fout/3, ForceCom/3
  Zshift/1 -> SwitchFz/2, SwitchFx/2, SwitchFy/2
  VelDiff-u/1 -> V^2-u/2, V-u/1
  V-u/1 -> V^2-u/1
  3x3/1 -> r x 3x1/2, r x 3x2/2, r x 3x3/2, A x 3x3/2
  Mz/1 -> Fout/6
  My/1 -> Fout/5
  Mx/1 -> Fout/4
  "r_{cg} x F"/1 -> Mx/1, My/1, Mz/1
  Fz-AFK/1 -> Fz-Sum/3
  Fz-A/1 -> Fz-Sum/2
  Fz-w/1 -> Fz-Sum/1
  Fx-AFK/1 -> Fx-Sum/3
  Fx-A/1 -> Fx-Sum/2
  Fx-V/1 -> Fx-Sum/1
  OrbitalVelocity/4(w-A) -> AccelDiff-w/1, Fz-AFK/1
  AccelDiff-w/1 -> Fz-A/1
  Vol/1 -> Fx-A/3, Fz-A/2, Fx-AFK/2, Fz-AFK/2, Fy-AFK/2, Fy-A/2
  AccelDiff-u/1 -> Fx-A/1
  V^2-w/1 -> Fz-w/1
  Density/1 -> Fx-V/3, Fx-V1/3, Fz-w/3, Fx-A/2, Fz-A/3, Fx-AFK/3, Fz-AFK/3, Fy-AFK/3, Fy-A/3
  half/1 -> Fx-V/2, Fx-V1/2, Fz-w/2
  V^2-u/1 -> Fx-V/1
  VelDiff-w/1 -> V^2-w/2, V-w/1
  OrbitalVelocity/2(w-V) -> VelDiff-w/1
  OrbitalVelocity/1(u-V) -> VelDiff-u/1
  Uz/1 -> VelDiff-w/2
  Ux/1 -> VelDiff-u/2
  Uy/1 -> VelDiff-v/2
  Add Vel/1 -> Ux/1, Uz/1, Uy/1
  "dot{U}z"/1 -> AccelDiff-w/2
  OrbitalVelocity/3(u-A) -> Fx-AFK/1, AccelDiff-u/1
  "dot{U}x"/1 -> AccelDiff-u/2
  "dot{U}y"/1 -> AccelDiff-v/2
  ShiftCg/1 -> OrbitalVelocity/1(Disp), Zshift/1
  Disp-sl/1 -> ShiftCg/2
  r x 3x3/1 -> ShiftCg/1, "r_{cg} x F"/1
  Rotation3/1(rot[3,1-3]) -> 3x3/3
  Rotation1/1(rot[1,1-3]) -> 3x3/1
  Rotation2/1(rot[2,1-3]) -> 3x3/2
  rot2/1 -> Rotation1/2(rot2), Rotation2/2(rot2), Rotation3/2(rot2)
  rot1/1 -> Rotation1/1(rot1), Rotation2/1(rot1), Rotation3/1(rot1)
  rot3/1 -> Rotation1/3(rot3), Rotation2/3(rot3)
  Disp-sr/1 -> rot1/1, rot2/1, rot3/1
  Disp/1 -> Disp-sr/1, Disp-sl/1
  Vel-sl/1 -> Add Vel/1
  Add Accel/1 -> "dot{U}x"/1, "dot{U}y"/1, "dot{U}z"/1
  Accel-sl/1 -> Add Accel/3
  "dot{w} x r2"/1 -> Add Accel/2
  Accel-sr/1 -> "dot{w} x r2"/1
  Accel/1 -> Accel-sr/1, Accel-sl/1
  r/1 -> w x r/2, "dot{w} x r2"/2, r x 3x3/1
  "Vel-sr "/1 -> w x r/1, w x w x r/1
  w x w x r/1 -> Add Accel/1
  w x r/1 -> w x w x r/2, Add Vel/2
  Vel/1 -> "Vel-sr "/1, Vel-sl/1

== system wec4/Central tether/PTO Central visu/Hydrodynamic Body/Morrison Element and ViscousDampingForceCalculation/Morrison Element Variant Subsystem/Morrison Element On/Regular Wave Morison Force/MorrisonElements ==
  r : Inport  Partition=on  PartitionDimension=1  PartitionWidth=1
  Vel : Inport  Port=2
  Accel : Inport  Port=3
  Disp : Inport  Port=4
  Area : Inport  Port=5  Partition=on  PartitionDimension=1  PartitionWidth=1
  Cd : Inport  Port=6  Partition=on  PartitionDimension=1  PartitionWidth=1
  Vol : Inport  Port=7  Partition=on  PartitionDimension=1  PartitionWidth=1
  Ca : Inport  Port=8  Partition=on  PartitionDimension=1  PartitionWidth=1
  Time : Inport  Port=9
  3x3 : Concatenate  NumInputs=3  Mode=Multidimensional array
  A x 3x3 : Product  Multiplication=Matrix(*)
  Accel-sl : Selector  InputPortWidth=6  IndexOptions=Index vector (dialog)  Indices=[1 2 3]  OutputSizes=1
  Accel-sr : Selector  InputPortWidth=6  IndexOptions=Index vector (dialog)  Indices=[4 5 6]  OutputSizes=1
  AccelDiff-u : Sum  Inputs=+-
  AccelDiff-v : Sum  Inputs=+-
  AccelDiff-w : Sum  Inputs=+-
  Add Accel : Sum  Inputs=+++
  Add Vel : Sum
  Ax : Selector  InputPortWidth=3  IndexOptions=Index vector (dialog)  Indices=[1]  OutputSizes=1
  Ay : Selector  InputPortWidth=3  IndexOptions=Index vector (dialog)  Indices=[2]  OutputSizes=1
  Az : Selector  InputPortWidth=3  IndexOptions=Index vector (dialog)  Indices=[3]  OutputSizes=1
  Cax : Selector  InputPortWidth=3  IndexOptions=Index vector (dialog)  Indices=[1]  OutputSizes=1
  Cay : Selector  InputPortWidth=3  IndexOptions=Index vector (dialog)  Indices=[2]  OutputSizes=1
  Caz : Selector  InputPortWidth=3  IndexOptions=Index vector (dialog)  Indices=[3]  OutputSizes=1
  Cdx : Selector  InputPortWidth=3  IndexOptions=Index vector (dialog)  Indices=[1]  OutputSizes=1
  Cdy : Selector  InputPortWidth=3  IndexOptions=Index vector (dialog)  Indices=[2]  OutputSizes=1
  Cdz : Selector  InputPortWidth=3  IndexOptions=Index vector (dialog)  Indices=[3]  OutputSizes=1
  Constant : Constant  Value=0
  Density : Constant  Value=simu.rho
  Disp-sl : Selector  InputPortWidth=6  IndexOptions=Index vector (dialog)  Indices=[1 2 3]  OutputSizes=1
  Disp-sr : Selector  InputPortWidth=6  IndexOptions=Index vector (dialog)  Indices=[4 5 6]  OutputSizes=1
  For Each : ForEach  DisableCoverage=on  IndexMode=One-based
  ForceCom : Concatenate  NumInputs=3  ConcatenateDimension=2
  Fout : Concatenate  NumInputs=6  Mode=Multidimensional array  ConcatenateDimension=2
  Fx-A : Product  Inputs=4
  Fx-AFK : Product  Inputs=3
  Fx-Sum : Sum  Inputs=+++
  Fx-V : Product  Inputs=5
  Fx-V1 : Product  Inputs=5
  Fy-A : Product  Inputs=4
  Fy-AFK : Product  Inputs=3
  Fy-Sum : Sum  Inputs=+++
  Fz-A : Product  Inputs=4
  Fz-AFK : Product  Inputs=3
  Fz-Sum : Sum  Inputs=+++
  Fz-w : Product  Inputs=5
  Mx : Selector  InputPortWidth=3  IndexOptions=Index vector (dialog)  Indices=[1]  OutputSizes=1
  My : Selector  InputPortWidth=3  IndexOptions=Index vector (dialog)  Indices=[2]  OutputSizes=1
  Mz : Selector  InputPortWidth=3  IndexOptions=Index vector (dialog)  Indices=[3]  OutputSizes=1
  OrbitalVelocity : Subsystem
  Rotation1 : Subsystem
  Rotation2 : Subsystem
  Rotation3 : Subsystem
  ShiftCg : Sum
  SwitchFx : Switch  Criteria=u2 > Threshold
  SwitchFy : Switch  Criteria=u2 > Threshold
  SwitchFz : Switch  Criteria=u2 > Threshold
  Ux : Selector  InputPortWidth=3  IndexOptions=Index vector (dialog)  Indices=[1]  OutputSizes=1
  Uy : Selector  InputPortWidth=3  IndexOptions=Index vector (dialog)  Indices=[2]  OutputSizes=1
  Uz : Selector  InputPortWidth=3  IndexOptions=Index vector (dialog)  Indices=[3]  OutputSizes=1
  V-u : Abs
  V-v : Abs
  V-w : Abs
  V^2-u : Product
  V^2-v : Product
  V^2-w : Product
  Vel-sl : Selector  InputPortWidth=6  IndexOptions=Index vector (dialog)  Indices=[1 2 3]  OutputSizes=1
  "Vel-sr " : Selector  InputPortWidth=6  IndexOptions=Index vector (dialog)  Indices=[4 5 6]  OutputSizes=1
  VelDiff-u : Sum  Inputs=+-
  VelDiff-v : Sum  Inputs=+-
  VelDiff-w : Sum  Inputs=+-
  Zshift : Selector  InputPortWidth=3  IndexOptions=Index vector (dialog)  Indices=[3]  OutputSizes=1
  abs-Area : Abs
  abs-Ca : Abs
  abs-Cd : Abs
  "dot{U}x" : Selector  InputPortWidth=3  IndexOptions=Index vector (dialog)  Indices=[1]  OutputSizes=1
  "dot{U}y" : Selector  InputPortWidth=3  IndexOptions=Index vector (dialog)  Indices=[2]  OutputSizes=1
  "dot{U}z" : Selector  InputPortWidth=3  IndexOptions=Index vector (dialog)  Indices=[3]  OutputSizes=1
  "dot{w} x r2" : vrlib/Utilities/Cross Product
  half : Constant  Value=1/2
  r x 3x1 : Product  Multiplication=Matrix(*)
  r x 3x2 : Product  Multiplication=Matrix(*)
  r x 3x3 : Product  Multiplication=Matrix(*)
  "r_{cg} x F" : vrlib/Utilities/Cross Product
  rot1 : Selector  InputPortWidth=3  IndexOptions=Index vector (dialog)  Indices=[1]  OutputSizes=1
  rot2 : Selector  InputPortWidth=3  IndexOptions=Index vector (dialog)  Indices=[2]  OutputSizes=1
  rot3 : Selector  InputPortWidth=3  IndexOptions=Index vector (dialog)  Indices=[3]  OutputSizes=1
  w x r : vrlib/Utilities/Cross Product
  w x w x r : vrlib/Utilities/Cross Product
  Force : Outport  PortDimensions=[1 6]  ConcatenationDimension=1
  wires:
  Time/1 -> OrbitalVelocity/2(Time)
  abs-Cd/1 -> r x 3x1/1
  abs-Ca/1 -> Caz/1, Cay/1, Cax/1
  V-w/1 -> V^2-w/1
  Constant/1 -> SwitchFx/1, SwitchFz/1, SwitchFy/1
  Fx-V1/1 -> Fy-Sum/1
  Fy-A/1 -> Fy-Sum/2
  Cay/1 -> Fy-A/4
  AccelDiff-v/1 -> Fy-A/1
  Fy-AFK/1 -> Fy-Sum/3
  Fy-Sum/1 -> SwitchFy/3
  SwitchFy/1 -> ForceCom/2, Fout/2
  Cdy/1 -> Fx-V1/4
  Ay/1 -> Fx-V1/5
  OrbitalVelocity/5(v-V) -> VelDiff-v/1
  VelDiff-v/1 -> V^2-v/2, V-v/1
  V-v/1 -> V^2-v/1
  V^2-v/1 -> Fx-V1/1
  OrbitalVelocity/6(v-A) -> Fy-AFK/1, AccelDiff-v/1
  r x 3x2/1 -> abs-Ca/1
  Ca/1 -> r x 3x2/1
  r x 3x1/1 -> Cdx/1, Cdz/1, Cdy/1
  Cd/1 -> abs-Cd/1
  Cax/1 -> Fx-A/4
  Caz/1 -> Fz-A/4
  Fout/1 -> Force/1
  ForceCom/1 -> "r_{cg} x F"/2
  abs-Area/1 -> Ax/1, Az/1, Ay/1
  A x 3x3/1 -> abs-Area/1
  Cdz/1 -> Fz-w/4
  Cdx/1 -> Fx-V/4
  Ax/1 -> Fx-V/5
  Area/1 -> A x 3x3/1
  Az/1 -> Fz-w/5
  Fz-Sum/1 -> SwitchFz/3
  Fx-Sum/1 -> SwitchFx/3
  SwitchFx/1 -> ForceCom/1, Fout/1
  SwitchFz/1 -> Fout/3, ForceCom/3
  Zshift/1 -> SwitchFz/2, SwitchFx/2, SwitchFy/2
  VelDiff-u/1 -> V^2-u/2, V-u/1
  V-u/1 -> V^2-u/1
  3x3/1 -> r x 3x1/2, r x 3x2/2, r x 3x3/2, A x 3x3/2
  Mz/1 -> Fout/6
  My/1 -> Fout/5
  Mx/1 -> Fout/4
  "r_{cg} x F"/1 -> Mx/1, My/1, Mz/1
  Fz-AFK/1 -> Fz-Sum/3
  Fz-A/1 -> Fz-Sum/2
  Fz-w/1 -> Fz-Sum/1
  Fx-AFK/1 -> Fx-Sum/3
  Fx-A/1 -> Fx-Sum/2
  Fx-V/1 -> Fx-Sum/1
  OrbitalVelocity/4(w-A) -> AccelDiff-w/1, Fz-AFK/1
  AccelDiff-w/1 -> Fz-A/1
  Vol/1 -> Fx-A/3, Fz-A/2, Fx-AFK/2, Fz-AFK/2, Fy-AFK/2, Fy-A/2
  AccelDiff-u/1 -> Fx-A/1
  V^2-w/1 -> Fz-w/1
  Density/1 -> Fx-V/3, Fx-V1/3, Fz-w/3, Fx-A/2, Fz-A/3, Fx-AFK/3, Fz-AFK/3, Fy-AFK/3, Fy-A/3
  half/1 -> Fx-V/2, Fx-V1/2, Fz-w/2
  V^2-u/1 -> Fx-V/1
  VelDiff-w/1 -> V^2-w/2, V-w/1
  OrbitalVelocity/2(w-V) -> VelDiff-w/1
  OrbitalVelocity/1(u-V) -> VelDiff-u/1
  Uz/1 -> VelDiff-w/2
  Ux/1 -> VelDiff-u/2
  Uy/1 -> VelDiff-v/2
  Add Vel/1 -> Ux/1, Uz/1, Uy/1
  "dot{U}z"/1 -> AccelDiff-w/2
  OrbitalVelocity/3(u-A) -> Fx-AFK/1, AccelDiff-u/1
  "dot{U}x"/1 -> AccelDiff-u/2
  "dot{U}y"/1 -> AccelDiff-v/2
  ShiftCg/1 -> OrbitalVelocity/1(Disp), Zshift/1
  Disp-sl/1 -> ShiftCg/2
  r x 3x3/1 -> ShiftCg/1, "r_{cg} x F"/1
  Rotation3/1(rot[3,1-3]) -> 3x3/3
  Rotation1/1(rot[1,1-3]) -> 3x3/1
  Rotation2/1(rot[2,1-3]) -> 3x3/2
  rot2/1 -> Rotation1/2(rot2), Rotation2/2(rot2), Rotation3/2(rot2)
  rot1/1 -> Rotation1/1(rot1), Rotation2/1(rot1), Rotation3/1(rot1)
  rot3/1 -> Rotation1/3(rot3), Rotation2/3(rot3)
  Disp-sr/1 -> rot1/1, rot2/1, rot3/1
  Disp/1 -> Disp-sr/1, Disp-sl/1
  Vel-sl/1 -> Add Vel/1
  Add Accel/1 -> "dot{U}x"/1, "dot{U}y"/1, "dot{U}z"/1
  Accel-sl/1 -> Add Accel/3
  "dot{w} x r2"/1 -> Add Accel/2
  Accel-sr/1 -> "dot{w} x r2"/1
  Accel/1 -> Accel-sr/1, Accel-sl/1
  r/1 -> w x r/2, "dot{w} x r2"/2, r x 3x3/1
  "Vel-sr "/1 -> w x r/1, w x w x r/1
  w x w x r/1 -> Add Accel/1
  w x r/1 -> w x w x r/2, Add Vel/2
  Vel/1 -> "Vel-sr "/1, Vel-sl/1

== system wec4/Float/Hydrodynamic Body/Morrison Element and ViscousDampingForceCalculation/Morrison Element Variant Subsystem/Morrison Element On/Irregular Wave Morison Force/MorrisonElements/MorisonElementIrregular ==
  Disp : Inport
  waves.kirr : Inport  Port=2  Partition=on  PartitionDimension=1  PartitionWidth=1
  waves.w : Inport  Port=3  Partition=on  PartitionDimension=1  PartitionWidth=1
  waves.A : Inport  Port=4  Partition=on  PartitionDimension=1  PartitionWidth=1
  waves.Phase : Inport  Port=5  Partition=on  PartitionDimension=1  PartitionWidth=1
  Time : Inport  Port=6
  For Each : ForEach  DisableCoverage=on  IndexMode=One-based
  MATLAB Function : MATLAB Function  TreatAsAtomicUnit=on
  gravity : Constant  Value=simu.g  VectorParams1D=off
  rampTime : Constant  Value=simu.rampTime  VectorParams1D=off
  waterDepth : Constant  Value=waves.waterDepth  VectorParams1D=off
  waveDirection : Constant  Value=waves.waveDir  VectorParams1D=off
  u-V : Outport  ConcatenationDimension=1
  w-V : Outport  Port=2  ConcatenationDimension=1
  x-A : Outport  Port=3  ConcatenationDimension=1
  w-A : Outport  Port=4  ConcatenationDimension=1
  v-V : Outport  Port=5  ConcatenationDimension=1
  y-A : Outport  Port=6  ConcatenationDimension=1
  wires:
  MATLAB Function/3(w) -> w-V/1
  MATLAB Function/4(xa) -> x-A/1
  MATLAB Function/6(za) -> w-A/1
  MATLAB Function/5(ya) -> y-A/1
  MATLAB Function/2(v) -> v-V/1
  Time/1 -> MATLAB Function/6(time)
  waves.kirr/1 -> MATLAB Function/2(waveNumber)
  MATLAB Function/1(u) -> u-V/1
  waves.Phase/1 -> MATLAB Function/5(phase)
  waves.A/1 -> MATLAB Function/4(waveAmp)
  waves.w/1 -> MATLAB Function/3(waveFreq)
  Disp/1 -> MATLAB Function/1(disp)
  rampTime/1 -> MATLAB Function/7(rampT)
  waveDirection/1 -> MATLAB Function/8(waveDir)
  waterDepth/1 -> MATLAB Function/9(waterDepth)
  gravity/1 -> MATLAB Function/10(g)

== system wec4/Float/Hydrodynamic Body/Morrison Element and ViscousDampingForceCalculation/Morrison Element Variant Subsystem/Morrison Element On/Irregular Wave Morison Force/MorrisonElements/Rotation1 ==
  rot1 : Inport
  rot2 : Inport  Port=2
  rot3 : Inport  Port=3
  2 : Product
  3 : Product  Inputs=3
  7 : Product
  8 : Product  Inputs=3
  Combine : Concatenate  NumInputs=3  Mode=Multidimensional array  ConcatenateDimension=2
  Trigonometric Function{,1..2,6,9,11} (6 alike) : Trigonometry  Operator=cos
  Trigonometric Function{3..5,7..8,10} (6 alike) : Trigonometry
  rot11 : Product
  rot12 : Sum
  rot13 : Sum  Inputs=+-
  rot[1,1-3] : Outport
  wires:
  rot13/1 -> Combine/3
  8/1 -> rot13/2
  7/1 -> rot13/1
  Trigonometric Function11/1 -> 8/3
  Trigonometric Function10/1 -> 8/2
  Trigonometric Function9/1 -> 8/1
  Trigonometric Function8/1 -> 7/2
  Trigonometric Function7/1 -> 7/1
  rot1/1 -> Trigonometric Function7/1, Trigonometric Function9/1, Trigonometric Function4/1, Trigonometric Function2/1
  rot3/1 -> Trigonometric Function8/1, Trigonometric Function11/1, Trigonometric Function6/1, Trigonometric Function3/1, Trigonometric Function1/1
  rot2/1 -> Trigonometric Function10/1, Trigonometric Function5/1, Trigonometric Function/1
  Combine/1 -> rot[1,1-3]/1
  rot12/1 -> Combine/2
  3/1 -> rot12/2
  2/1 -> rot12/1
  Trigonometric Function6/1 -> 3/3
  Trigonometric Function5/1 -> 3/2
  Trigonometric Function4/1 -> 3/1
  Trigonometric Function3/1 -> 2/2
  Trigonometric Function2/1 -> 2/1
  rot11/1 -> Combine/1
  Trigonometric Function1/1 -> rot11/2
  Trigonometric Function/1 -> rot11/1

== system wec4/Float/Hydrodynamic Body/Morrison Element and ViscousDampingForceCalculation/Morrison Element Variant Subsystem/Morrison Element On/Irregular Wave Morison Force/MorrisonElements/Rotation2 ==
  rot1 : Inport
  rot2 : Inport  Port=2
  rot3 : Inport  Port=3
  2 : Product
  3 : Product  Inputs=3
  7 : Product
  8 : Product  Inputs=3
  Combine : Concatenate  NumInputs=3  Mode=Multidimensional array  ConcatenateDimension=2
  Gain : Gain  Gain=-1
  Trigonometric Function{,2..3,8..9} (5 alike) : Trigonometry  Operator=cos
  Trigonometric Function{1,4..7,10..11} (7 alike) : Trigonometry
  rot11 : Product
  rot12 : Sum  Inputs=+-
  rot13 : Sum
  rot[2,1-3] : Outport
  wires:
  Gain/1 -> rot11/1
  rot13/1 -> Combine/3
  8/1 -> rot13/2
  7/1 -> rot13/1
  Trigonometric Function11/1 -> 8/3
  Trigonometric Function10/1 -> 8/2
  Trigonometric Function9/1 -> 8/1
  Trigonometric Function8/1 -> 7/2
  Trigonometric Function7/1 -> 7/1
  rot1/1 -> Trigonometric Function7/1, Trigonometric Function9/1, Trigonometric Function4/1, Trigonometric Function2/1
  rot3/1 -> Trigonometric Function8/1, Trigonometric Function11/1, Trigonometric Function6/1, Trigonometric Function3/1, Trigonometric Function1/1
  rot2/1 -> Trigonometric Function10/1, Trigonometric Function5/1, Trigonometric Function/1
  Combine/1 -> rot[2,1-3]/1
  rot12/1 -> Combine/2
  3/1 -> rot12/2
  2/1 -> rot12/1
  Trigonometric Function6/1 -> 3/3
  Trigonometric Function5/1 -> 3/2
  Trigonometric Function4/1 -> 3/1
  Trigonometric Function3/1 -> 2/2
  Trigonometric Function2/1 -> 2/1
  rot11/1 -> Combine/1
  Trigonometric Function1/1 -> rot11/2
  Trigonometric Function/1 -> Gain/1

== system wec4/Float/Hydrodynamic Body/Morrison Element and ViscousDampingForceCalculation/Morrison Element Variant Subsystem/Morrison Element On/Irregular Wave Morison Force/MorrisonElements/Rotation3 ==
  rot1 : Inport
  rot2 : Inport  Port=2
  2 : Product
  7 : Product
  Combine : Concatenate  NumInputs=3  Mode=Multidimensional array  ConcatenateDimension=2
  Gain1 : Gain  Gain=-1
  TrigFun1 : Trigonometry
  TrigFun2 : Trigonometry
  TrigFun3 : Trigonometry  Operator=cos
  TrigFun4 : Trigonometry  Operator=cos
  TrigFun5 : Trigonometry  Operator=cos
  rot[3,1-3] : Outport
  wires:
  Gain1/1 -> 2/1
  TrigFun2/1 -> Gain1/1
  7/1 -> Combine/3
  rot1/1 -> TrigFun4/1, TrigFun2/1
  TrigFun5/1 -> 7/2
  TrigFun4/1 -> 7/1
  rot2/1 -> TrigFun1/1, TrigFun3/1, TrigFun5/1
  Combine/1 -> rot[3,1-3]/1
  2/1 -> Combine/2
  TrigFun3/1 -> 2/2
  TrigFun1/1 -> Combine/1
